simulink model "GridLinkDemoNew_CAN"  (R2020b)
settings: Solver=FixedStepDiscrete  StartTime=0.0  StopTime=inf  RelTol=1e-3  EnableMultiTasking=on
InitFcn:
  | clc
  | close all
  | f_mod = 50000;
  | f_mod1 = 50*1e3; %[12 24 36 48 72 84 96 144]*1e3; %[18 36 48 72 84 96 144]*1e3;%
  | 
  | 
  | %%
  | 
  | 
  |             Tmod1 = 1/f_mod1;
  |             Tmod = 1/f_mod;
  |             Tc = Tmod1;
  |             Tsw=Tc;
  | 
  | warning off
  | f_sig = 60;
  | 
  | U_ac = 10;
  | U_dc = 20;
  | Ts= 0.01*Tsw;
  | 
  | Fc=50000
  | Fc1=1000
  | 
  | 
  | CounterCut_Outer=2000
  | 
  | 
  | INNER_PWM=1000
  | OUTER_PWM=50000
undefined symbols (not defined in the file): A, ADCIN0, ADCIN1, ADCINA0, ADCINB0, bit, Compare, conversion, DCAEVT1, DCAEVT1FILT, Digital, Down, ended, Event, Filtered, GPTRIP1SEL, GPTRIP2SEL, hex2dec, identifier, input, Module, Newinv, of, Single, SPS_EMT_TAPAS_2018b, Standard, start, Trip, TZ1, TZ2, Up, version, Zone
libraries: tiiqmathlib x63, c2802xlib x25, c2837xDlib x5, c280xlib x5, c28xdmclib x2, svdutilitieslib x1, c2000lib x1, canmsglib x1, simulink x1
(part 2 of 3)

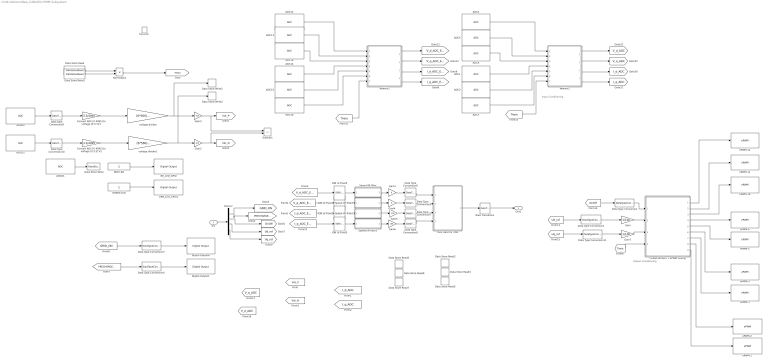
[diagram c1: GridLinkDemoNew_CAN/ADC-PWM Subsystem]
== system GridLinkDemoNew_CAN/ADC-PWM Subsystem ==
  note: Output Conditioning
  note: Input Conditioning
  In1 : Inport
  function : TriggerPort  TriggerType=function-call  VariantControl=Variant
  ADC1 : c2802xlib/ADC  blkParamProc=C2000_Type4  ADCModule=A  samplingMode=Single sample mode  ADCResolution=12-bit (Single-ended input)  useSOC1=SOC12  useSOC2=SOC0_SOC1  SOCAcquisitionWindow=13  SOCTriggerSource=ePWM12_ADCSOCA  SOCInterruptTrigger=No ADCINT  Ts=-1  dType=uint16  postInterrupt=off  interruptSel=ADCINT1  ADCINTContinuous=on  endma=off  chdma=1  conv1=ADCINA0  conv2=ADCINA0 and ADCINB0  conv1_Type4=ADCIN3  conv2_Type4=ADCIN0 and ADCIN1
  ADC12 : c2802xlib/ADC  blkParamProc=C2000_Type4  ADCModule=A  samplingMode=Single sample mode  ADCResolution=12-bit (Single-ended input)  useSOC1=SOC0  useSOC2=SOC0_SOC1  SOCAcquisitionWindow=13  SOCTriggerSource=ePWM12_ADCSOCA  SOCInterruptTrigger=No ADCINT  Ts=-1  dType=uint16  postInterrupt=off  interruptSel=ADCINT1  ADCINTContinuous=on  endma=off  chdma=1  conv1=ADCINA0  conv2=ADCINA0 and ADCINB0  conv1_Type4=ADCIN0  conv2_Type4=ADCIN0 and ADCIN1
  ADC13 : c2802xlib/ADC  blkParamProc=C2000_Type4  ADCModule=A  samplingMode=Single sample mode  ADCResolution=12-bit (Single-ended input)  useSOC1=SOC15  useSOC2=SOC0_SOC1  SOCAcquisitionWindow=13  SOCTriggerSource=ePWM12_ADCSOCA  SOCInterruptTrigger=No ADCINT  Ts=-1  dType=uint16  postInterrupt=on  interruptSel=ADCINT1  ADCINTContinuous=off  endma=off  chdma=1  conv1=ADCINA0  conv2=ADCINA0 and ADCINB0  conv1_Type4=ADCIN1  conv2_Type4=ADCIN0 and ADCIN1
  ADC14 : c2802xlib/ADC  blkParamProc=C2000_Type4  ADCModule=B  samplingMode=Single sample mode  ADCResolution=12-bit (Single-ended input)  useSOC1=SOC3  useSOC2=SOC0_SOC1  SOCAcquisitionWindow=13  SOCTriggerSource=ePWM12_ADCSOCA  SOCInterruptTrigger=No ADCINT  Ts=-1  dType=uint16  postInterrupt=off  interruptSel=ADCINT1  ADCINTContinuous=on  endma=off  chdma=1  conv1=ADCINA0  conv2=ADCINA0 and ADCINB0  conv1_Type4=ADCIN2  conv2_Type4=ADCIN0 and ADCIN1
  ADC15 : c2802xlib/ADC  blkParamProc=C2000_Type4  ADCModule=D  samplingMode=Single sample mode  ADCResolution=12-bit (Single-ended input)  useSOC1=SOC4  useSOC2=SOC0_SOC1  SOCAcquisitionWindow=13  SOCTriggerSource=ePWM12_ADCSOCA  SOCInterruptTrigger=No ADCINT  Ts=-1  dType=uint16  postInterrupt=off  interruptSel=ADCINT1  ADCINTContinuous=on  endma=off  chdma=1  conv1=ADCINA0  conv2=ADCINA0 and ADCINB0  conv1_Type4=ADCIN14  conv2_Type4=ADCIN0 and ADCIN1
  ADC16 : c2802xlib/ADC  blkParamProc=C2000_Type4  ADCModule=C  samplingMode=Single sample mode  ADCResolution=12-bit (Single-ended input)  useSOC1=SOC5  useSOC2=SOC0_SOC1  SOCAcquisitionWindow=13  SOCTriggerSource=ePWM12_ADCSOCA  SOCInterruptTrigger=No ADCINT  Ts=-1  dType=uint16  postInterrupt=off  interruptSel=ADCINT1  ADCINTContinuous=on  endma=off  chdma=1  conv1=ADCINA0  conv2=ADCINA0 and ADCINB0  conv1_Type4=ADCIN2  conv2_Type4=ADCIN0 and ADCIN1
  ADC19 : c2802xlib/ADC  blkParamProc=C2000_Type4  ADCModule=B  samplingMode=Single sample mode  ADCResolution=12-bit (Single-ended input)  useSOC1=SOC2  useSOC2=SOC0_SOC1  SOCAcquisitionWindow=13  SOCTriggerSource=ePWM12_ADCSOCA  SOCInterruptTrigger=No ADCINT  Ts=-1  dType=uint16  postInterrupt=off  interruptSel=ADCINT1  ADCINTContinuous=on  endma=off  chdma=1  conv1=ADCINA0  conv2=ADCINA0 and ADCINB0  conv1_Type4=ADCIN1  conv2_Type4=ADCIN0 and ADCIN1
  ADC2 : c2802xlib/ADC  blkParamProc=C2000_Type4  ADCModule=B  samplingMode=Single sample mode  ADCResolution=12-bit (Single-ended input)  useSOC1=SOC13  useSOC2=SOC0_SOC1  SOCAcquisitionWindow=13  SOCTriggerSource=ePWM12_ADCSOCA  SOCInterruptTrigger=No ADCINT  Ts=-1  dType=uint16  postInterrupt=off  interruptSel=ADCINT1  ADCINTContinuous=on  endma=off  chdma=1  conv1=ADCINA0  conv2=ADCINA0 and ADCINB0  conv1_Type4=ADCIN0  conv2_Type4=ADCIN0 and ADCIN1
  ADC3 : c2802xlib/ADC  blkParamProc=C2000_Type4  ADCModule=D  samplingMode=Single sample mode  ADCResolution=12-bit (Single-ended input)  useSOC1=SOC2  useSOC2=SOC0_SOC1  SOCAcquisitionWindow=13  SOCTriggerSource=ePWM12_ADCSOCA  SOCInterruptTrigger=No ADCINT  Ts=-1  dType=uint16  postInterrupt=off  interruptSel=ADCINT1  ADCINTContinuous=off  endma=off  chdma=1  conv1=ADCINA0  conv2=ADCINA0 and ADCINB0  conv1_Type4=ADCIN4  conv2_Type4=ADCIN0 and ADCIN1
  ADC4 : c2802xlib/ADC  blkParamProc=C2000_Type4  ADCModule=A  samplingMode=Single sample mode  ADCResolution=12-bit (Single-ended input)  useSOC1=SOC9  useSOC2=SOC0_SOC1  SOCAcquisitionWindow=13  SOCTriggerSource=ePWM12_ADCSOCA  SOCInterruptTrigger=No ADCINT  Ts=-1  dType=uint16  postInterrupt=off  interruptSel=ADCINT1  ADCINTContinuous=on  endma=off  chdma=1  conv1=ADCINA0  conv2=ADCINA0 and ADCINB0  conv1_Type4=ADCIN5  conv2_Type4=ADCIN0 and ADCIN1
  ADC5 : c2802xlib/ADC  blkParamProc=C2000_Type4  ADCModule=B  samplingMode=Single sample mode  ADCResolution=12-bit (Single-ended input)  useSOC1=SOC10  useSOC2=SOC0_SOC1  SOCAcquisitionWindow=13  SOCTriggerSource=ePWM12_ADCSOCA  SOCInterruptTrigger=No ADCINT  Ts=-1  dType=uint16  postInterrupt=off  interruptSel=ADCINT1  ADCINTContinuous=on  endma=off  chdma=1  conv1=ADCINA0  conv2=ADCINA0 and ADCINB0  conv1_Type4=ADCIN4  conv2_Type4=ADCIN0 and ADCIN1
  ADC6 : c2802xlib/ADC  blkParamProc=C2000_Type4  ADCModule=D  samplingMode=Single sample mode  ADCResolution=12-bit (Single-ended input)  useSOC1=SOC11  useSOC2=SOC0_SOC1  SOCAcquisitionWindow=13  SOCTriggerSource=ePWM12_ADCSOCA  SOCInterruptTrigger=No ADCINT  Ts=-1  dType=uint16  postInterrupt=off  interruptSel=ADCINT1  ADCINTContinuous=on  endma=off  chdma=1  conv1=ADCINA0  conv2=ADCINA0 and ADCINB0  conv1_Type4=ADCIN5  conv2_Type4=ADCIN0 and ADCIN1
  ADCD0 : c2802xlib/ADC  blkParamProc=C2000_Type4  ADCModule=D  samplingMode=Single sample mode  ADCResolution=12-bit (Single-ended input)  useSOC1=SOC6  useSOC2=SOC0_SOC1  SOCAcquisitionWindow=13  SOCTriggerSource=ePWM12_ADCSOCA  SOCInterruptTrigger=No ADCINT  Ts=-1  dType=uint16  postInterrupt=off  interruptSel=ADCINT1  ADCINTContinuous=off  endma=off  chdma=1  conv1=ADCINA0  conv2=ADCINA0 and ADCINB0  conv1_Type4=ADCIN0  conv2_Type4=ADCIN0 and ADCIN1
  ADCD1 : c2802xlib/ADC  blkParamProc=C2000_Type4  ADCModule=D  samplingMode=Single sample mode  ADCResolution=12-bit (Single-ended input)  useSOC1=SOC7  useSOC2=SOC0_SOC1  SOCAcquisitionWindow=13  SOCTriggerSource=ePWM12_ADCSOCA  SOCInterruptTrigger=No ADCINT  Ts=-1  dType=uint16  postInterrupt=off  interruptSel=ADCINT1  ADCINTContinuous=off  endma=off  chdma=1  conv1=ADCINA0  conv2=ADCINA0 and ADCINB0  conv1_Type4=ADCIN1  conv2_Type4=ADCIN0 and ADCIN1
  ADCD2 : c2802xlib/ADC  blkParamProc=C2000_Type4  ADCModule=D  samplingMode=Single sample mode  ADCResolution=12-bit (Single-ended input)  useSOC1=SOC8  useSOC2=SOC0_SOC1  SOCAcquisitionWindow=13  SOCTriggerSource=ePWM12_ADCSOCA  SOCInterruptTrigger=No ADCINT  Ts=-1  dType=uint16  postInterrupt=off  interruptSel=ADCINT2  ADCINTContinuous=off  endma=off  chdma=1  conv1=ADCINA0  conv2=ADCINA0 and ADCINB0  conv1_Type4=ADCIN2  conv2_Type4=ADCIN0 and ADCIN1
  Convert ADC [0 4095] to voltage [0 3.3] V : Gain  Gain=3.3/4095  ParamDataTypeStr=Inherit: Inherit from 'Gain'  OutDataTypeStr=single
  Convert ADC [0 4095] to voltage [0 3.3] V1 : Gain  Gain=3.3/4095  ParamDataTypeStr=Inherit: Inherit from 'Gain'  OutDataTypeStr=single
  Data Store Read : DataStoreRead  DataStoreName=Counter
  Data Store Read1 : DataStoreRead  DataStoreName=CounterCut
  Data Store Read2 : DataStoreRead  DataStoreName=I_o_C
  Data Store Read3 : DataStoreRead  DataStoreName=I_s_C
  Data Store Read4 : DataStoreRead  DataStoreName=I_s_B
  Data Store Read5 : DataStoreRead  DataStoreName=I_s_A
  Data Store Read6 : DataStoreRead  DataStoreName=I_o_B
  Data Store Read7 : DataStoreRead  DataStoreName=I_o_A
  Data Store Write : DataStoreWrite  DataStoreName=Temp_P1
  Data Store Write1 : DataStoreWrite  DataStoreName=VdcP
  Data Store Write2 : DataStoreWrite  DataStoreName=VdcN
  Data Type Conversion : DataTypeConversion  OutDataTypeStr=boolean
  Data Type Conversion{1,5..11} (8 alike) : DataTypeConversion  OutDataTypeStr=single
  Data Type Conversion3 : DataTypeConversion  OutDataTypeStr=boolean
  Data Type Conversion4 : DataTypeConversion  OutDataTypeStr=boolean
  Demux : Demux
  Digital Output1 : c2837xDlib/Digital Output  GPIO_Number=GPIO64~GPIO71  GPIO_Bit0=off  GPIO_BIT0_Toggle=on  GPIO_Bit1=off  GPIO_BIT1_Toggle=on  GPIO_Bit2=off  GPIO_BIT2_Toggle=off  GPIO_Bit3=off  GPIO_BIT3_Toggle=off  GPIO_Bit4=off  GPIO_BIT4_Toggle=off  GPIO_Bit5=off  GPIO_BIT5_Toggle=off  GPIO_Bit6=off  GPIO_BIT6_Toggle=off  GPIO_Bit7=on  GPIO_BIT7_Toggle=off
  Digital Output6 : c2837xDlib/Digital Output  GPIO_Number=GPIO56~GPIO63  GPIO_Bit0=off  GPIO_BIT0_Toggle=off  GPIO_Bit1=on  GPIO_BIT1_Toggle=off  GPIO_Bit2=off  GPIO_BIT2_Toggle=off  GPIO_Bit3=off  GPIO_BIT3_Toggle=off  GPIO_Bit4=off  GPIO_BIT4_Toggle=off  GPIO_Bit5=off  GPIO_BIT5_Toggle=on  GPIO_Bit6=off  GPIO_BIT6_Toggle=off  GPIO_Bit7=off  GPIO_BIT7_Toggle=on
  GREEN LED : Constant  OutDataTypeStr=boolean  SampleTime=-1
  GRN_LED_GPIO1 : c2837xDlib/Digital Output  GPIO_Number=GPIO112~GPIO119  GPIO_Bit0=off  GPIO_BIT0_Toggle=on  GPIO_Bit1=off  GPIO_BIT1_Toggle=on  GPIO_Bit2=on  GPIO_BIT2_Toggle=off  GPIO_Bit3=off  GPIO_BIT3_Toggle=off  GPIO_Bit4=off  GPIO_BIT4_Toggle=off  GPIO_Bit5=off  GPIO_BIT5_Toggle=on  GPIO_Bit6=off  GPIO_BIT6_Toggle=off  GPIO_Bit7=off  GPIO_BIT7_Toggle=on
  Gain : Gain  Gain=1/100
  Gain1 : Gain
  Gain2 : Gain  Gain=100  ParamDataTypeStr=Inherit: Inherit from 'Gain'
  Gain3 : Gain  Gain=100  ParamDataTypeStr=Inherit: Inherit from 'Gain'
  Gain4 : Gain
  Gain5 : Gain  Gain=100
  Gain6 : Gain  Gain=100
  Gain7 : Gain  Gain=1/100
  IQN to Float{1..3,5} (4 alike) : tiiqmathlib/IQN to Float
  InvPark/SVGen + ePWM scaling : Subsystem
  Newinv1 : Subsystem  AncestorBlock=SPS_EMT_TAPAS_2018b/Newinv  TreatAsAtomicUnit=on
  Newinv2 : Subsystem  AncestorBlock=SPS_EMT_TAPAS_2018b/Newinv  TreatAsAtomicUnit=on
  Normalize1 : Product  Inputs=*/
  Pack data for CAN : Subsystem
  RD_LED_GPIO : c2837xDlib/Digital Output  GPIO_Number=GPIO112~GPIO119  GPIO_Bit0=off  GPIO_BIT0_Toggle=on  GPIO_Bit1=on  GPIO_BIT1_Toggle=off  GPIO_Bit2=off  GPIO_BIT2_Toggle=on  GPIO_Bit3=off  GPIO_BIT3_Toggle=off  GPIO_Bit4=off  GPIO_BIT4_Toggle=off  GPIO_Bit5=off  GPIO_BIT5_Toggle=off  GPIO_Bit6=off  GPIO_BIT6_Toggle=on  GPIO_Bit7=off  GPIO_BIT7_Toggle=on
  RED LED : Constant  OutDataTypeStr=boolean  SampleTime=-1
  Rate Transition1 : RateTransition
  Speed IIR filter : Subsystem
  Speed IIR filter1 : Subsystem
  Speed IIR filter2 : Subsystem
  Speed IIR filter3 : Subsystem
  Subtract : Sum  Inputs=+-
  "ePWM-1 " : c2802xlib/ePWM  PwmType=C2000_Type4  useModule=ePWM1  ePWMxLINKTBPRD=Not Linked  periodUnits=Clock cycles  timerSource=Specify via dialog  timerPeriod_clk=INNER_PWM  timerPeriod_sec=0.0001  tbshadow=Counter equals to zero  countingMode=Up-Down  phaseActiveEnable=Set counter to phase value specified via dialog  phaseDirection=Count up after sync  phaseActive=0  synchronizationEnable=off  dcaevt1Sync=off  dcbevt1Sync=off  synchronizationOption=Disable  perSynchronizationOption=Counter equals to period (CTR=PRD)  clockPrescale=1  HSclockPrescale=1  enswap=off  ePWMxAStatus=on  ePWMxAactionLogic1=Do nothing  ePWMxAactionLogic2=Do nothing  ePWMxAactionLogic3=Clear  ePWMxAactionLogic4=Set  ePWMxAactionLogic5=Do nothing  ePWMxAactionLogic6=Do nothing  ePWMxACSFenable=off  ePWMxACSFvalue=Forcing disable  ePWMxASFreload=Immediate  ePWMxBStatus=off  ePWMxBactionLogic1=Do nothing  ePWMxBactionLogic2=Do nothing  ePWMxBactionLogic3=Clear  ePWMxBactionLogic4=Set  ePWMxBactionLogic5=Do nothing  ePWMxBactionLogic6=Do nothing  ePWMxBCSFenable=off  ePWMxBCSFvalue=Forcing disable  ePWMxBSFreload=Immediate  ePWNxBOutWay=off  ePWMxLINKCMPA=Not Linked  CMPAUnits=Clock cycles  CMPASource=Input port  CMPAValue_per=50  CMPAValue_clk=0  enCMPAshadow=Counter equals to zero (CTR=Zero)  ePWMxLINKCMPB=Not Linked  CMPBUnits=Clock cycles  CMPBSource=Specify via dialog  CMPBValue_per=50  CMPBValue_clk=32000  enCMPBshadow=Counter equals to zero (CTR=Zero)  ePWMxLINKCMPC=Not Linked  CMPCUnits=Clock cycles  CMPCSource=Specify via dialog  CMPCValue_per=50  CMPCValue_clk=32000  enCMPCshadow=Counter equals to zero (CTR=Zero)  ePWMxLINKCMPD=Not Linked  CMPDUnits=Clock cycles  CMPDSource=Specify via dialog  CMPDValue_per=50  CMPDValue_clk=32000  enCMPDshadow=Counter equals to zero (CTR=Zero)  enableDBePWMxA=on  enableDBePWMxB=on  enhalfcycle=off  DBpolarity=Active high complementary (AHC)  DBedgeDelay=Positive  DBSource_ePWMxA=ePWMxA  DBSource_ePWMxB=ePWMxA  DBPeriodUnits=Clock cycles  DBperiodSource=Specify via dialog  REDperiod=2  FEDperiod=2  REDperiod_sec=0  FEDperiod_sec=0  LoadModeDBRED=Immediate without using shadow  LoadModeDBFED=Immediate without using shadow  adcstartModuleA=off  adcrequestEventA=First event  adcstartEventA=Digital Compare Module A Event 1 start of conversion (DCAEVT1.soc)  adcstartEventA_type2=Counter equals to period (CTR=PRD)  adcstartModuleB=off  adcrequestEventB=First event  adcstartEventB=Counter equals to zero (CTR=Zero)  adcstartEventB_type2=Counter equals to zero (CTR=Zero)  intEn=off  intPrd=First event  intSel=Counter equals to zero (CTR=Zero)  intSel_type2=Counter equals to zero (CTR=Zero)  hrpe=off  enHRPWM=off  HRPWM_LoadMode=Counter equals to period (CTR=PRD)  HRPWM_CTLMode=Duty or Period control mode  HRPWM_EDGMode=Both edge  hrpeb=off  enHRPWMB=off  HRPWM_LoadModeB=Counter equals to zero (CTR=ZERO)  HRPWM_CTLModeB=Duty or Period control mode  HRPWM_EDGModeB=Both edge  enHRDBRED=off  enHRDBFED=off  enSFO=on  enautoconv=on  chopperEnable=off  chopperFrequency=1  chopperFirstwidth=1  chopperDuty=12.5%  tripZonesource=Specify via dialog  tzselOSHT1=off  tzselOSHT2=off  tzselOSHT3=off  tzselOSHDCAEV1=off  tzselOSHDCBEV1=off  tzselCBC1=off  tzselCBC2=off  tzselCBC3=off  tzselCBCDCAEV2=off  tzselCBCDCBEV2=off  tzselOSHT4=off  tzselOSHT5=off  tzselOSHT6=off  tzselCBC4=off  tzselCBC5=off  tzselCBC6=off  enTzOstIntr=off  enTzCbcIntr=off  enTzDCAEVT1Intr=off  enTzDCAEVT2Intr=off  enTzDCBEVT1Intr=off  enTzDCBEVT2Intr=off  ePWMxAforced=No action  ePWMxBforced=No action  DCAEVT1forced=No action  DCBEVT1forced=No action  DCAEVT2forced=No action  DCBEVT2forced=No action  dcah=Trip Zone 1 input (TZ1)  dcal=Trip Zone 2 input (TZ2)  dcbh=Trip Zone 1 input (TZ1)  dcbl=Trip Zone 2 input (TZ2)  dcah_type2=GPTRIP1SEL/(TZ1)  dcal_type2=GPTRIP2SEL/(TZ2)  dcbh_type2=GPTRIP1SEL/(TZ1)  dcbl_type2=GPTRIP2SEL/(TZ2)  gendcaevt1=Event disabled  gendcaevt2=Event disabled  gendcbevt1=Event disabled  gendcbevt2=Event disabled  dcaevt1src=DCAEVT1 with sync  dcaevt2src=DCAEVT2 with sync  dcbevt1src=DCBEVT1 with sync  dcbevt2src=DCBEVT2 with sync  pulsesel=Counter equals to zero (CTR=Zero)  blankinv=off  blankoffset=0  blankwidth=0  evsrcsel=Filtered version of DCAEVT1 (DCAEVT1FILT)  encape=off
  ePWM-10 : c2802xlib/ePWM  PwmType=C2000_Type4  useModule=ePWM10  ePWMxLINKTBPRD=Not Linked  periodUnits=Clock cycles  timerSource=Specify via dialog  timerPeriod_clk=OUTER_PWM  timerPeriod_sec=0.0001  tbshadow=Counter equals to zero  countingMode=Up-Down  phaseActiveEnable=Set counter to phase value specified via dialog  phaseDirection=Count up after sync  phaseActive=0  synchronizationEnable=off  dcaevt1Sync=off  dcbevt1Sync=off  synchronizationOption=Disable  perSynchronizationOption=Counter equals to period (CTR=PRD)  clockPrescale=1  HSclockPrescale=1  enswap=off  ePWMxAStatus=on  ePWMxAactionLogic1=Do nothing  ePWMxAactionLogic2=Do nothing  ePWMxAactionLogic3=Clear  ePWMxAactionLogic4=Set  ePWMxAactionLogic5=Do nothing  ePWMxAactionLogic6=Do nothing  ePWMxACSFenable=off  ePWMxACSFvalue=Forcing disable  ePWMxASFreload=Immediate  ePWMxBStatus=off  ePWMxBactionLogic1=Do nothing  ePWMxBactionLogic2=Do nothing  ePWMxBactionLogic3=Clear  ePWMxBactionLogic4=Set  ePWMxBactionLogic5=Do nothing  ePWMxBactionLogic6=Do nothing  ePWMxBCSFenable=off  ePWMxBCSFvalue=Forcing disable  ePWMxBSFreload=Immediate  ePWNxBOutWay=off  ePWMxLINKCMPA=Not Linked  CMPAUnits=Clock cycles  CMPASource=Input port  CMPAValue_per=50  CMPAValue_clk=0  enCMPAshadow=Counter equals to zero (CTR=Zero)  ePWMxLINKCMPB=Not Linked  CMPBUnits=Clock cycles  CMPBSource=Specify via dialog  CMPBValue_per=50  CMPBValue_clk=32000  enCMPBshadow=Counter equals to zero (CTR=Zero)  ePWMxLINKCMPC=Not Linked  CMPCUnits=Clock cycles  CMPCSource=Specify via dialog  CMPCValue_per=50  CMPCValue_clk=32000  enCMPCshadow=Counter equals to zero (CTR=Zero)  ePWMxLINKCMPD=Not Linked  CMPDUnits=Clock cycles  CMPDSource=Specify via dialog  CMPDValue_per=50  CMPDValue_clk=32000  enCMPDshadow=Counter equals to zero (CTR=Zero)  enableDBePWMxA=on  enableDBePWMxB=on  enhalfcycle=off  DBpolarity=Active high complementary (AHC)  DBedgeDelay=Positive  DBSource_ePWMxA=ePWMxA  DBSource_ePWMxB=ePWMxA  DBPeriodUnits=Clock cycles  DBperiodSource=Specify via dialog  REDperiod=25  FEDperiod=25  REDperiod_sec=0  FEDperiod_sec=0  LoadModeDBRED=Immediate without using shadow  LoadModeDBFED=Immediate without using shadow  adcstartModuleA=off  adcrequestEventA=First event  adcstartEventA=Digital Compare Module A Event 1 start of conversion (DCAEVT1.soc)  adcstartEventA_type2=Counter equals to period (CTR=PRD)  adcstartModuleB=off  adcrequestEventB=First event  adcstartEventB=Counter equals to zero (CTR=Zero)  adcstartEventB_type2=Counter equals to zero (CTR=Zero)  intEn=off  intPrd=First event  intSel=Counter equals to zero (CTR=Zero)  intSel_type2=Counter equals to zero (CTR=Zero)  hrpe=off  enHRPWM=off  HRPWM_LoadMode=Counter equals to period (CTR=PRD)  HRPWM_CTLMode=Duty or Period control mode  HRPWM_EDGMode=Both edge  hrpeb=off  enHRPWMB=off  HRPWM_LoadModeB=Counter equals to zero (CTR=ZERO)  HRPWM_CTLModeB=Duty or Period control mode  HRPWM_EDGModeB=Both edge  enHRDBRED=off  enHRDBFED=off  enSFO=on  enautoconv=on  chopperEnable=off  chopperFrequency=1  chopperFirstwidth=1  chopperDuty=12.5%  tripZonesource=Specify via dialog  tzselOSHT1=off  tzselOSHT2=off  tzselOSHT3=off  tzselOSHDCAEV1=off  tzselOSHDCBEV1=off  tzselCBC1=off  tzselCBC2=off  tzselCBC3=off  tzselCBCDCAEV2=off  tzselCBCDCBEV2=off  tzselOSHT4=off  tzselOSHT5=off  tzselOSHT6=off  tzselCBC4=off  tzselCBC5=off  tzselCBC6=off  enTzOstIntr=off  enTzCbcIntr=off  enTzDCAEVT1Intr=off  enTzDCAEVT2Intr=off  enTzDCBEVT1Intr=off  enTzDCBEVT2Intr=off  ePWMxAforced=No action  ePWMxBforced=No action  DCAEVT1forced=No action  DCBEVT1forced=No action  DCAEVT2forced=No action  DCBEVT2forced=No action  dcah=Trip Zone 1 input (TZ1)  dcal=Trip Zone 2 input (TZ2)  dcbh=Trip Zone 1 input (TZ1)  dcbl=Trip Zone 2 input (TZ2)  dcah_type2=GPTRIP1SEL/(TZ1)  dcal_type2=GPTRIP2SEL/(TZ2)  dcbh_type2=GPTRIP1SEL/(TZ1)  dcbl_type2=GPTRIP2SEL/(TZ2)  gendcaevt1=Event disabled  gendcaevt2=Event disabled  gendcbevt1=Event disabled  gendcbevt2=Event disabled  dcaevt1src=DCAEVT1 with sync  dcaevt2src=DCAEVT2 with sync  dcbevt1src=DCBEVT1 with sync  dcbevt2src=DCBEVT2 with sync  pulsesel=Counter equals to zero (CTR=Zero)  blankinv=off  blankoffset=0  blankwidth=0  evsrcsel=Filtered version of DCAEVT1 (DCAEVT1FILT)  encape=off
  ePWM-11 : c2802xlib/ePWM  PwmType=C2000_Type4  useModule=ePWM11  ePWMxLINKTBPRD=Not Linked  periodUnits=Clock cycles  timerSource=Specify via dialog  timerPeriod_clk=OUTER_PWM  timerPeriod_sec=0.0001  tbshadow=Counter equals to zero  countingMode=Up-Down  phaseActiveEnable=Set counter to phase value specified via dialog  phaseDirection=Count up after sync  phaseActive=0  synchronizationEnable=off  dcaevt1Sync=off  dcbevt1Sync=off  synchronizationOption=Pass through (EPWMxSYNCI or SWFSYNC)  perSynchronizationOption=Counter equals to period (CTR=PRD)  clockPrescale=1  HSclockPrescale=1  enswap=off  ePWMxAStatus=on  ePWMxAactionLogic1=Do nothing  ePWMxAactionLogic2=Do nothing  ePWMxAactionLogic3=Clear  ePWMxAactionLogic4=Set  ePWMxAactionLogic5=Do nothing  ePWMxAactionLogic6=Do nothing  ePWMxACSFenable=off  ePWMxACSFvalue=Forcing disable  ePWMxASFreload=Immediate  ePWMxBStatus=off  ePWMxBactionLogic1=Do nothing  ePWMxBactionLogic2=Do nothing  ePWMxBactionLogic3=Clear  ePWMxBactionLogic4=Set  ePWMxBactionLogic5=Do nothing  ePWMxBactionLogic6=Do nothing  ePWMxBCSFenable=off  ePWMxBCSFvalue=Forcing disable  ePWMxBSFreload=Immediate  ePWNxBOutWay=off  ePWMxLINKCMPA=Not Linked  CMPAUnits=Clock cycles  CMPASource=Input port  CMPAValue_per=50  CMPAValue_clk=0  enCMPAshadow=Counter equals to zero (CTR=Zero)  ePWMxLINKCMPB=Not Linked  CMPBUnits=Clock cycles  CMPBSource=Specify via dialog  CMPBValue_per=50  CMPBValue_clk=32000  enCMPBshadow=Counter equals to zero (CTR=Zero)  ePWMxLINKCMPC=Not Linked  CMPCUnits=Clock cycles  CMPCSource=Specify via dialog  CMPCValue_per=50  CMPCValue_clk=32000  enCMPCshadow=Counter equals to zero (CTR=Zero)  ePWMxLINKCMPD=Not Linked  CMPDUnits=Clock cycles  CMPDSource=Specify via dialog  CMPDValue_per=50  CMPDValue_clk=32000  enCMPDshadow=Counter equals to zero (CTR=Zero)  enableDBePWMxA=on  enableDBePWMxB=on  enhalfcycle=off  DBpolarity=Active high complementary (AHC)  DBedgeDelay=Positive  DBSource_ePWMxA=ePWMxA  DBSource_ePWMxB=ePWMxA  DBPeriodUnits=Clock cycles  DBperiodSource=Specify via dialog  REDperiod=25  FEDperiod=25  REDperiod_sec=0  FEDperiod_sec=0  LoadModeDBRED=Immediate without using shadow  LoadModeDBFED=Immediate without using shadow  adcstartModuleA=off  adcrequestEventA=First event  adcstartEventA=Digital Compare Module A Event 1 start of conversion (DCAEVT1.soc)  adcstartEventA_type2=Counter equals to period (CTR=PRD)  adcstartModuleB=off  adcrequestEventB=First event  adcstartEventB=Counter equals to zero (CTR=Zero)  adcstartEventB_type2=Counter equals to zero (CTR=Zero)  intEn=off  intPrd=First event  intSel=Counter equals to zero (CTR=Zero)  intSel_type2=Counter equals to zero (CTR=Zero)  hrpe=off  enHRPWM=off  HRPWM_LoadMode=Counter equals to period (CTR=PRD)  HRPWM_CTLMode=Duty or Period control mode  HRPWM_EDGMode=Both edge  hrpeb=off  enHRPWMB=off  HRPWM_LoadModeB=Counter equals to zero (CTR=ZERO)  HRPWM_CTLModeB=Duty or Period control mode  HRPWM_EDGModeB=Both edge  enHRDBRED=off  enHRDBFED=off  enSFO=on  enautoconv=on  chopperEnable=off  chopperFrequency=1  chopperFirstwidth=1  chopperDuty=12.5%  tripZonesource=Specify via dialog  tzselOSHT1=off  tzselOSHT2=off  tzselOSHT3=off  tzselOSHDCAEV1=off  tzselOSHDCBEV1=off  tzselCBC1=off  tzselCBC2=off  tzselCBC3=off  tzselCBCDCAEV2=off  tzselCBCDCBEV2=off  tzselOSHT4=off  tzselOSHT5=off  tzselOSHT6=off  tzselCBC4=off  tzselCBC5=off  tzselCBC6=off  enTzOstIntr=off  enTzCbcIntr=off  enTzDCAEVT1Intr=off  enTzDCAEVT2Intr=off  enTzDCBEVT1Intr=off  enTzDCBEVT2Intr=off  ePWMxAforced=No action  ePWMxBforced=No action  DCAEVT1forced=No action  DCBEVT1forced=No action  DCAEVT2forced=No action  DCBEVT2forced=No action  dcah=Trip Zone 1 input (TZ1)  dcal=Trip Zone 2 input (TZ2)  dcbh=Trip Zone 1 input (TZ1)  dcbl=Trip Zone 2 input (TZ2)  dcah_type2=GPTRIP1SEL/(TZ1)  dcal_type2=GPTRIP2SEL/(TZ2)  dcbh_type2=GPTRIP1SEL/(TZ1)  dcbl_type2=GPTRIP2SEL/(TZ2)  gendcaevt1=Event disabled  gendcaevt2=Event disabled  gendcbevt1=Event disabled  gendcbevt2=Event disabled  dcaevt1src=DCAEVT1 with sync  dcaevt2src=DCAEVT2 with sync  dcbevt1src=DCBEVT1 with sync  dcbevt2src=DCBEVT2 with sync  pulsesel=Counter equals to zero (CTR=Zero)  blankinv=off  blankoffset=0  blankwidth=0  evsrcsel=Filtered version of DCAEVT1 (DCAEVT1FILT)  encape=off
  ePWM-12 : c2802xlib/ePWM  PwmType=C2000_Type4  useModule=ePWM12  ePWMxLINKTBPRD=Not Linked  periodUnits=Clock cycles  timerSource=Specify via dialog  timerPeriod_clk=OUTER_PWM  timerPeriod_sec=0.0001  tbshadow=Counter equals to zero  countingMode=Up-Down  phaseActiveEnable=Disable  phaseDirection=Count down after sync  phaseActive=0  synchronizationEnable=off  dcaevt1Sync=off  dcbevt1Sync=off  synchronizationOption=Counter equals to zero (CTR=Zero)  perSynchronizationOption=Counter equals to period (CTR=PRD)  clockPrescale=1  HSclockPrescale=1  enswap=off  ePWMxAStatus=on  ePWMxAactionLogic1=Do nothing  ePWMxAactionLogic2=Do nothing  ePWMxAactionLogic3=Clear  ePWMxAactionLogic4=Set  ePWMxAactionLogic5=Do nothing  ePWMxAactionLogic6=Do nothing  ePWMxACSFenable=off  ePWMxACSFvalue=Forcing disable  ePWMxASFreload=Immediate  ePWMxBStatus=off  ePWMxBactionLogic1=Do nothing  ePWMxBactionLogic2=Do nothing  ePWMxBactionLogic3=Clear  ePWMxBactionLogic4=Set  ePWMxBactionLogic5=Do nothing  ePWMxBactionLogic6=Do nothing  ePWMxBCSFenable=off  ePWMxBCSFvalue=Forcing disable  ePWMxBSFreload=Immediate  ePWNxBOutWay=off  ePWMxLINKCMPA=Not Linked  CMPAUnits=Clock cycles  CMPASource=Input port  CMPAValue_per=50  CMPAValue_clk=0  enCMPAshadow=Counter equals to zero (CTR=Zero)  ePWMxLINKCMPB=Not Linked  CMPBUnits=Clock cycles  CMPBSource=Specify via dialog  CMPBValue_per=50  CMPBValue_clk=32000  enCMPBshadow=Counter equals to zero (CTR=Zero)  ePWMxLINKCMPC=Not Linked  CMPCUnits=Clock cycles  CMPCSource=Specify via dialog  CMPCValue_per=50  CMPCValue_clk=32000  enCMPCshadow=Counter equals to zero (CTR=Zero)  ePWMxLINKCMPD=Not Linked  CMPDUnits=Clock cycles  CMPDSource=Specify via dialog  CMPDValue_per=50  CMPDValue_clk=32000  enCMPDshadow=Counter equals to zero (CTR=Zero)  enableDBePWMxA=on  enableDBePWMxB=on  enhalfcycle=on  DBpolarity=Active high complementary (AHC)  DBedgeDelay=Positive  DBSource_ePWMxA=ePWMxA  DBSource_ePWMxB=ePWMxA  DBPeriodUnits=Clock cycles  DBperiodSource=Specify via dialog  REDperiod=25  FEDperiod=25  REDperiod_sec=0  FEDperiod_sec=0  LoadModeDBRED=Immediate without using shadow  LoadModeDBFED=Immediate without using shadow  adcstartModuleA=on  adcrequestEventA=First event  adcstartEventA=Digital Compare Module A Event 1 start of conversion (DCAEVT1.soc)  adcstartEventA_type2=Counter equals to period (CTR=PRD)  adcstartModuleB=off  adcrequestEventB=First event  adcstartEventB=Counter equals to zero (CTR=Zero)  adcstartEventB_type2=Counter equals to zero (CTR=Zero)  intEn=off  intPrd=First event  intSel=Counter equals to zero (CTR=Zero)  intSel_type2=Counter equals to zero (CTR=Zero)  hrpe=off  enHRPWM=off  HRPWM_LoadMode=Counter equals to period (CTR=PRD)  HRPWM_CTLMode=Duty or Period control mode  HRPWM_EDGMode=Both edge  hrpeb=off  enHRPWMB=off  HRPWM_LoadModeB=Counter equals to zero (CTR=ZERO)  HRPWM_CTLModeB=Duty or Period control mode  HRPWM_EDGModeB=Both edge  enHRDBRED=off  enHRDBFED=off  enSFO=on  enautoconv=on  chopperEnable=off  chopperFrequency=1  chopperFirstwidth=1  chopperDuty=12.5%  tripZonesource=Specify via dialog  tzselOSHT1=off  tzselOSHT2=off  tzselOSHT3=off  tzselOSHDCAEV1=off  tzselOSHDCBEV1=off  tzselCBC1=off  tzselCBC2=off  tzselCBC3=off  tzselCBCDCAEV2=off  tzselCBCDCBEV2=off  tzselOSHT4=off  tzselOSHT5=off  tzselOSHT6=off  tzselCBC4=off  tzselCBC5=off  tzselCBC6=off  enTzOstIntr=off  enTzCbcIntr=off  enTzDCAEVT1Intr=off  enTzDCAEVT2Intr=off  enTzDCBEVT1Intr=off  enTzDCBEVT2Intr=off  ePWMxAforced=No action  ePWMxBforced=No action  DCAEVT1forced=No action  DCBEVT1forced=No action  DCAEVT2forced=No action  DCBEVT2forced=No action  dcah=Trip Zone 1 input (TZ1)  dcal=Trip Zone 2 input (TZ2)  dcbh=Trip Zone 1 input (TZ1)  dcbl=Trip Zone 2 input (TZ2)  dcah_type2=GPTRIP1SEL/(TZ1)  dcal_type2=GPTRIP2SEL/(TZ2)  dcbh_type2=GPTRIP1SEL/(TZ1)  dcbl_type2=GPTRIP2SEL/(TZ2)  gendcaevt1=Event disabled  gendcaevt2=Event disabled  gendcbevt1=Event disabled  gendcbevt2=Event disabled  dcaevt1src=DCAEVT1 with sync  dcaevt2src=DCAEVT2 with sync  dcbevt1src=DCBEVT1 with sync  dcbevt2src=DCBEVT2 with sync  pulsesel=Counter equals to zero (CTR=Zero)  blankinv=off  blankoffset=0  blankwidth=0  evsrcsel=Filtered version of DCAEVT1 (DCAEVT1FILT)  encape=off
  "ePWM-2 " : c2802xlib/ePWM  PwmType=C2000_Type4  useModule=ePWM2  ePWMxLINKTBPRD=Not Linked  periodUnits=Clock cycles  timerSource=Specify via dialog  timerPeriod_clk=INNER_PWM  timerPeriod_sec=0.0001  tbshadow=Counter equals to zero  countingMode=Up-Down  phaseActiveEnable=Set counter to phase value specified via dialog  phaseDirection=Count up after sync  phaseActive=0  synchronizationEnable=off  dcaevt1Sync=off  dcbevt1Sync=off  synchronizationOption=Disable  perSynchronizationOption=Counter equals to period (CTR=PRD)  clockPrescale=1  HSclockPrescale=1  enswap=off  ePWMxAStatus=on  ePWMxAactionLogic1=Do nothing  ePWMxAactionLogic2=Do nothing  ePWMxAactionLogic3=Clear  ePWMxAactionLogic4=Set  ePWMxAactionLogic5=Do nothing  ePWMxAactionLogic6=Do nothing  ePWMxACSFenable=off  ePWMxACSFvalue=Forcing disable  ePWMxASFreload=Immediate  ePWMxBStatus=off  ePWMxBactionLogic1=Do nothing  ePWMxBactionLogic2=Do nothing  ePWMxBactionLogic3=Clear  ePWMxBactionLogic4=Set  ePWMxBactionLogic5=Do nothing  ePWMxBactionLogic6=Do nothing  ePWMxBCSFenable=off  ePWMxBCSFvalue=Forcing disable  ePWMxBSFreload=Immediate  ePWNxBOutWay=off  ePWMxLINKCMPA=Not Linked  CMPAUnits=Clock cycles  CMPASource=Input port  CMPAValue_per=50  CMPAValue_clk=0  enCMPAshadow=Counter equals to zero (CTR=Zero)  ePWMxLINKCMPB=Not Linked  CMPBUnits=Clock cycles  CMPBSource=Specify via dialog  CMPBValue_per=50  CMPBValue_clk=32000  enCMPBshadow=Counter equals to zero (CTR=Zero)  ePWMxLINKCMPC=Not Linked  CMPCUnits=Clock cycles  CMPCSource=Specify via dialog  CMPCValue_per=50  CMPCValue_clk=32000  enCMPCshadow=Counter equals to zero (CTR=Zero)  ePWMxLINKCMPD=Not Linked  CMPDUnits=Clock cycles  CMPDSource=Specify via dialog  CMPDValue_per=50  CMPDValue_clk=32000  enCMPDshadow=Counter equals to zero (CTR=Zero)  enableDBePWMxA=on  enableDBePWMxB=on  enhalfcycle=off  DBpolarity=Active high complementary (AHC)  DBedgeDelay=Positive  DBSource_ePWMxA=ePWMxA  DBSource_ePWMxB=ePWMxA  DBPeriodUnits=Clock cycles  DBperiodSource=Specify via dialog  REDperiod=2  FEDperiod=2  REDperiod_sec=0  FEDperiod_sec=0  LoadModeDBRED=Immediate without using shadow  LoadModeDBFED=Immediate without using shadow  adcstartModuleA=off  adcrequestEventA=First event  adcstartEventA=Digital Compare Module A Event 1 start of conversion (DCAEVT1.soc)  adcstartEventA_type2=Counter equals to period (CTR=PRD)  adcstartModuleB=off  adcrequestEventB=First event  adcstartEventB=Counter equals to zero (CTR=Zero)  adcstartEventB_type2=Counter equals to zero (CTR=Zero)  intEn=off  intPrd=First event  intSel=Counter equals to zero (CTR=Zero)  intSel_type2=Counter equals to zero (CTR=Zero)  hrpe=off  enHRPWM=off  HRPWM_LoadMode=Counter equals to period (CTR=PRD)  HRPWM_CTLMode=Duty or Period control mode  HRPWM_EDGMode=Both edge  hrpeb=off  enHRPWMB=off  HRPWM_LoadModeB=Counter equals to zero (CTR=ZERO)  HRPWM_CTLModeB=Duty or Period control mode  HRPWM_EDGModeB=Both edge  enHRDBRED=off  enHRDBFED=off  enSFO=on  enautoconv=on  chopperEnable=off  chopperFrequency=1  chopperFirstwidth=1  chopperDuty=12.5%  tripZonesource=Specify via dialog  tzselOSHT1=off  tzselOSHT2=off  tzselOSHT3=off  tzselOSHDCAEV1=off  tzselOSHDCBEV1=off  tzselCBC1=off  tzselCBC2=off  tzselCBC3=off  tzselCBCDCAEV2=off  tzselCBCDCBEV2=off  tzselOSHT4=off  tzselOSHT5=off  tzselOSHT6=off  tzselCBC4=off  tzselCBC5=off  tzselCBC6=off  enTzOstIntr=off  enTzCbcIntr=off  enTzDCAEVT1Intr=off  enTzDCAEVT2Intr=off  enTzDCBEVT1Intr=off  enTzDCBEVT2Intr=off  ePWMxAforced=No action  ePWMxBforced=No action  DCAEVT1forced=No action  DCBEVT1forced=No action  DCAEVT2forced=No action  DCBEVT2forced=No action  dcah=Trip Zone 1 input (TZ1)  dcal=Trip Zone 2 input (TZ2)  dcbh=Trip Zone 1 input (TZ1)  dcbl=Trip Zone 2 input (TZ2)  dcah_type2=GPTRIP1SEL/(TZ1)  dcal_type2=GPTRIP2SEL/(TZ2)  dcbh_type2=GPTRIP1SEL/(TZ1)  dcbl_type2=GPTRIP2SEL/(TZ2)  gendcaevt1=Event disabled  gendcaevt2=Event disabled  gendcbevt1=Event disabled  gendcbevt2=Event disabled  dcaevt1src=DCAEVT1 with sync  dcaevt2src=DCAEVT2 with sync  dcbevt1src=DCBEVT1 with sync  dcbevt2src=DCBEVT2 with sync  pulsesel=Counter equals to zero (CTR=Zero)  blankinv=off  blankoffset=0  blankwidth=0  evsrcsel=Filtered version of DCAEVT1 (DCAEVT1FILT)  encape=off
  ePWM-3 : c2802xlib/ePWM  PwmType=C2000_Type4  useModule=ePWM3  ePWMxLINKTBPRD=Not Linked  periodUnits=Clock cycles  timerSource=Specify via dialog  timerPeriod_clk=INNER_PWM  timerPeriod_sec=0.0001  tbshadow=Counter equals to zero  countingMode=Up-Down  phaseActiveEnable=Set counter to phase value specified via dialog  phaseDirection=Count up after sync  phaseActive=0  synchronizationEnable=off  dcaevt1Sync=off  dcbevt1Sync=off  synchronizationOption=Pass through (EPWMxSYNCI or SWFSYNC)  perSynchronizationOption=Counter equals to period (CTR=PRD)  clockPrescale=1  HSclockPrescale=1  enswap=off  ePWMxAStatus=on  ePWMxAactionLogic1=Do nothing  ePWMxAactionLogic2=Do nothing  ePWMxAactionLogic3=Clear  ePWMxAactionLogic4=Set  ePWMxAactionLogic5=Do nothing  ePWMxAactionLogic6=Do nothing  ePWMxACSFenable=off  ePWMxACSFvalue=Forcing disable  ePWMxASFreload=Immediate  ePWMxBStatus=off  ePWMxBactionLogic1=Do nothing  ePWMxBactionLogic2=Do nothing  ePWMxBactionLogic3=Clear  ePWMxBactionLogic4=Set  ePWMxBactionLogic5=Do nothing  ePWMxBactionLogic6=Do nothing  ePWMxBCSFenable=off  ePWMxBCSFvalue=Forcing disable  ePWMxBSFreload=Immediate  ePWNxBOutWay=off  ePWMxLINKCMPA=Not Linked  CMPAUnits=Clock cycles  CMPASource=Input port  CMPAValue_per=50  CMPAValue_clk=0  enCMPAshadow=Counter equals to zero (CTR=Zero)  ePWMxLINKCMPB=Not Linked  CMPBUnits=Clock cycles  CMPBSource=Specify via dialog  CMPBValue_per=50  CMPBValue_clk=32000  enCMPBshadow=Counter equals to zero (CTR=Zero)  ePWMxLINKCMPC=Not Linked  CMPCUnits=Clock cycles  CMPCSource=Specify via dialog  CMPCValue_per=50  CMPCValue_clk=32000  enCMPCshadow=Counter equals to zero (CTR=Zero)  ePWMxLINKCMPD=Not Linked  CMPDUnits=Clock cycles  CMPDSource=Specify via dialog  CMPDValue_per=50  CMPDValue_clk=32000  enCMPDshadow=Counter equals to zero (CTR=Zero)  enableDBePWMxA=on  enableDBePWMxB=on  enhalfcycle=off  DBpolarity=Active high complementary (AHC)  DBedgeDelay=Positive  DBSource_ePWMxA=ePWMxA  DBSource_ePWMxB=ePWMxA  DBPeriodUnits=Clock cycles  DBperiodSource=Specify via dialog  REDperiod=2  FEDperiod=2  REDperiod_sec=0  FEDperiod_sec=0  LoadModeDBRED=Immediate without using shadow  LoadModeDBFED=Immediate without using shadow  adcstartModuleA=off  adcrequestEventA=First event  adcstartEventA=Digital Compare Module A Event 1 start of conversion (DCAEVT1.soc)  adcstartEventA_type2=Counter equals to period (CTR=PRD)  adcstartModuleB=off  adcrequestEventB=First event  adcstartEventB=Counter equals to zero (CTR=Zero)  adcstartEventB_type2=Counter equals to zero (CTR=Zero)  intEn=off  intPrd=First event  intSel=Counter equals to zero (CTR=Zero)  intSel_type2=Counter equals to zero (CTR=Zero)  hrpe=off  enHRPWM=off  HRPWM_LoadMode=Counter equals to period (CTR=PRD)  HRPWM_CTLMode=Duty or Period control mode  HRPWM_EDGMode=Both edge  hrpeb=off  enHRPWMB=off  HRPWM_LoadModeB=Counter equals to zero (CTR=ZERO)  HRPWM_CTLModeB=Duty or Period control mode  HRPWM_EDGModeB=Both edge  enHRDBRED=off  enHRDBFED=off  enSFO=on  enautoconv=on  chopperEnable=off  chopperFrequency=1  chopperFirstwidth=1  chopperDuty=12.5%  tripZonesource=Specify via dialog  tzselOSHT1=off  tzselOSHT2=off  tzselOSHT3=off  tzselOSHDCAEV1=off  tzselOSHDCBEV1=off  tzselCBC1=off  tzselCBC2=off  tzselCBC3=off  tzselCBCDCAEV2=off  tzselCBCDCBEV2=off  tzselOSHT4=off  tzselOSHT5=off  tzselOSHT6=off  tzselCBC4=off  tzselCBC5=off  tzselCBC6=off  enTzOstIntr=off  enTzCbcIntr=off  enTzDCAEVT1Intr=off  enTzDCAEVT2Intr=off  enTzDCBEVT1Intr=off  enTzDCBEVT2Intr=off  ePWMxAforced=No action  ePWMxBforced=No action  DCAEVT1forced=No action  DCBEVT1forced=No action  DCAEVT2forced=No action  DCBEVT2forced=No action  dcah=Trip Zone 1 input (TZ1)  dcal=Trip Zone 2 input (TZ2)  dcbh=Trip Zone 1 input (TZ1)  dcbl=Trip Zone 2 input (TZ2)  dcah_type2=GPTRIP1SEL/(TZ1)  dcal_type2=GPTRIP2SEL/(TZ2)  dcbh_type2=GPTRIP1SEL/(TZ1)  dcbl_type2=GPTRIP2SEL/(TZ2)  gendcaevt1=Event disabled  gendcaevt2=Event disabled  gendcbevt1=Event disabled  gendcbevt2=Event disabled  dcaevt1src=DCAEVT1 with sync  dcaevt2src=DCAEVT2 with sync  dcbevt1src=DCBEVT1 with sync  dcbevt2src=DCBEVT2 with sync  pulsesel=Counter equals to zero (CTR=Zero)  blankinv=off  blankoffset=0  blankwidth=0  evsrcsel=Filtered version of DCAEVT1 (DCAEVT1FILT)  encape=off
  ePWM-4 : c2802xlib/ePWM  PwmType=C2000_Type4  useModule=ePWM4  ePWMxLINKTBPRD=Not Linked  periodUnits=Clock cycles  timerSource=Specify via dialog  timerPeriod_clk=INNER_PWM  timerPeriod_sec=0.0001  tbshadow=Counter equals to zero  countingMode=Up-Down  phaseActiveEnable=Set counter to phase value specified via dialog  phaseDirection=Count up after sync  phaseActive=0  synchronizationEnable=off  dcaevt1Sync=off  dcbevt1Sync=off  synchronizationOption=Pass through (EPWMxSYNCI or SWFSYNC)  perSynchronizationOption=Counter equals to period (CTR=PRD)  clockPrescale=1  HSclockPrescale=1  enswap=off  ePWMxAStatus=on  ePWMxAactionLogic1=Do nothing  ePWMxAactionLogic2=Do nothing  ePWMxAactionLogic3=Clear  ePWMxAactionLogic4=Set  ePWMxAactionLogic5=Do nothing  ePWMxAactionLogic6=Do nothing  ePWMxACSFenable=off  ePWMxACSFvalue=Forcing disable  ePWMxASFreload=Immediate  ePWMxBStatus=off  ePWMxBactionLogic1=Do nothing  ePWMxBactionLogic2=Do nothing  ePWMxBactionLogic3=Clear  ePWMxBactionLogic4=Set  ePWMxBactionLogic5=Do nothing  ePWMxBactionLogic6=Do nothing  ePWMxBCSFenable=off  ePWMxBCSFvalue=Forcing disable  ePWMxBSFreload=Immediate  ePWNxBOutWay=off  ePWMxLINKCMPA=Not Linked  CMPAUnits=Clock cycles  CMPASource=Input port  CMPAValue_per=50  CMPAValue_clk=0  enCMPAshadow=Counter equals to zero (CTR=Zero)  ePWMxLINKCMPB=Not Linked  CMPBUnits=Clock cycles  CMPBSource=Specify via dialog  CMPBValue_per=50  CMPBValue_clk=32000  enCMPBshadow=Counter equals to zero (CTR=Zero)  ePWMxLINKCMPC=Not Linked  CMPCUnits=Clock cycles  CMPCSource=Specify via dialog  CMPCValue_per=50  CMPCValue_clk=32000  enCMPCshadow=Counter equals to zero (CTR=Zero)  ePWMxLINKCMPD=Not Linked  CMPDUnits=Clock cycles  CMPDSource=Specify via dialog  CMPDValue_per=50  CMPDValue_clk=32000  enCMPDshadow=Counter equals to zero (CTR=Zero)  enableDBePWMxA=on  enableDBePWMxB=on  enhalfcycle=off  DBpolarity=Active high complementary (AHC)  DBedgeDelay=Positive  DBSource_ePWMxA=ePWMxA  DBSource_ePWMxB=ePWMxA  DBPeriodUnits=Clock cycles  DBperiodSource=Specify via dialog  REDperiod=2  FEDperiod=2  REDperiod_sec=0  FEDperiod_sec=0  LoadModeDBRED=Immediate without using shadow  LoadModeDBFED=Immediate without using shadow  adcstartModuleA=off  adcrequestEventA=First event  adcstartEventA=Digital Compare Module A Event 1 start of conversion (DCAEVT1.soc)  adcstartEventA_type2=Counter equals to period (CTR=PRD)  adcstartModuleB=off  adcrequestEventB=First event  adcstartEventB=Counter equals to zero (CTR=Zero)  adcstartEventB_type2=Counter equals to zero (CTR=Zero)  intEn=off  intPrd=First event  intSel=Counter equals to zero (CTR=Zero)  intSel_type2=Counter equals to zero (CTR=Zero)  hrpe=off  enHRPWM=off  HRPWM_LoadMode=Counter equals to period (CTR=PRD)  HRPWM_CTLMode=Duty or Period control mode  HRPWM_EDGMode=Both edge  hrpeb=off  enHRPWMB=off  HRPWM_LoadModeB=Counter equals to zero (CTR=ZERO)  HRPWM_CTLModeB=Duty or Period control mode  HRPWM_EDGModeB=Both edge  enHRDBRED=off  enHRDBFED=off  enSFO=on  enautoconv=on  chopperEnable=off  chopperFrequency=1  chopperFirstwidth=1  chopperDuty=12.5%  tripZonesource=Specify via dialog  tzselOSHT1=off  tzselOSHT2=off  tzselOSHT3=off  tzselOSHDCAEV1=off  tzselOSHDCBEV1=off  tzselCBC1=off  tzselCBC2=off  tzselCBC3=off  tzselCBCDCAEV2=off  tzselCBCDCBEV2=off  tzselOSHT4=off  tzselOSHT5=off  tzselOSHT6=off  tzselCBC4=off  tzselCBC5=off  tzselCBC6=off  enTzOstIntr=off  enTzCbcIntr=off  enTzDCAEVT1Intr=off  enTzDCAEVT2Intr=off  enTzDCBEVT1Intr=off  enTzDCBEVT2Intr=off  ePWMxAforced=No action  ePWMxBforced=No action  DCAEVT1forced=No action  DCBEVT1forced=No action  DCAEVT2forced=No action  DCBEVT2forced=No action  dcah=Trip Zone 1 input (TZ1)  dcal=Trip Zone 2 input (TZ2)  dcbh=Trip Zone 1 input (TZ1)  dcbl=Trip Zone 2 input (TZ2)  dcah_type2=GPTRIP1SEL/(TZ1)  dcal_type2=GPTRIP2SEL/(TZ2)  dcbh_type2=GPTRIP1SEL/(TZ1)  dcbl_type2=GPTRIP2SEL/(TZ2)  gendcaevt1=Event disabled  gendcaevt2=Event disabled  gendcbevt1=Event disabled  gendcbevt2=Event disabled  dcaevt1src=DCAEVT1 with sync  dcaevt2src=DCAEVT2 with sync  dcbevt1src=DCBEVT1 with sync  dcbevt2src=DCBEVT2 with sync  pulsesel=Counter equals to zero (CTR=Zero)  blankinv=off  blankoffset=0  blankwidth=0  evsrcsel=Filtered version of DCAEVT1 (DCAEVT1FILT)  encape=off
  ePWM-5 : c2802xlib/ePWM  PwmType=C2000_Type4  useModule=ePWM5  ePWMxLINKTBPRD=Not Linked  periodUnits=Clock cycles  timerSource=Specify via dialog  timerPeriod_clk=INNER_PWM  timerPeriod_sec=0.0001  tbshadow=Counter equals to zero  countingMode=Up-Down  phaseActiveEnable=Disable  phaseDirection=Count up after sync  phaseActive=0  synchronizationEnable=off  dcaevt1Sync=off  dcbevt1Sync=off  synchronizationOption=Counter equals to zero (CTR=Zero)  perSynchronizationOption=Counter equals to period (CTR=PRD)  clockPrescale=1  HSclockPrescale=1  enswap=off  ePWMxAStatus=on  ePWMxAactionLogic1=Do nothing  ePWMxAactionLogic2=Do nothing  ePWMxAactionLogic3=Clear  ePWMxAactionLogic4=Set  ePWMxAactionLogic5=Do nothing  ePWMxAactionLogic6=Do nothing  ePWMxACSFenable=off  ePWMxACSFvalue=Forcing disable  ePWMxASFreload=Immediate  ePWMxBStatus=off  ePWMxBactionLogic1=Do nothing  ePWMxBactionLogic2=Do nothing  ePWMxBactionLogic3=Clear  ePWMxBactionLogic4=Set  ePWMxBactionLogic5=Do nothing  ePWMxBactionLogic6=Do nothing  ePWMxBCSFenable=off  ePWMxBCSFvalue=Forcing disable  ePWMxBSFreload=Immediate  ePWNxBOutWay=off  ePWMxLINKCMPA=Not Linked  CMPAUnits=Clock cycles  CMPASource=Input port  CMPAValue_per=50  CMPAValue_clk=0  enCMPAshadow=Counter equals to zero (CTR=Zero)  ePWMxLINKCMPB=Not Linked  CMPBUnits=Clock cycles  CMPBSource=Specify via dialog  CMPBValue_per=50  CMPBValue_clk=32000  enCMPBshadow=Counter equals to zero (CTR=Zero)  ePWMxLINKCMPC=Not Linked  CMPCUnits=Clock cycles  CMPCSource=Specify via dialog  CMPCValue_per=50  CMPCValue_clk=32000  enCMPCshadow=Counter equals to zero (CTR=Zero)  ePWMxLINKCMPD=Not Linked  CMPDUnits=Clock cycles  CMPDSource=Specify via dialog  CMPDValue_per=50  CMPDValue_clk=32000  enCMPDshadow=Counter equals to zero (CTR=Zero)  enableDBePWMxA=on  enableDBePWMxB=on  enhalfcycle=on  DBpolarity=Active high complementary (AHC)  DBedgeDelay=Positive  DBSource_ePWMxA=ePWMxA  DBSource_ePWMxB=ePWMxA  DBPeriodUnits=Clock cycles  DBperiodSource=Specify via dialog  REDperiod=2  FEDperiod=2  REDperiod_sec=0  FEDperiod_sec=0  LoadModeDBRED=Immediate without using shadow  LoadModeDBFED=Immediate without using shadow  adcstartModuleA=off  adcrequestEventA=First event  adcstartEventA=Digital Compare Module A Event 1 start of conversion (DCAEVT1.soc)  adcstartEventA_type2=Counter equals to period (CTR=PRD)  adcstartModuleB=off  adcrequestEventB=First event  adcstartEventB=Counter equals to zero (CTR=Zero)  adcstartEventB_type2=Counter equals to zero (CTR=Zero)  intEn=off  intPrd=First event  intSel=Counter equals to zero (CTR=Zero)  intSel_type2=Counter equals to zero (CTR=Zero)  hrpe=off  enHRPWM=off  HRPWM_LoadMode=Counter equals to period (CTR=PRD)  HRPWM_CTLMode=Duty or Period control mode  HRPWM_EDGMode=Both edge  hrpeb=off  enHRPWMB=off  HRPWM_LoadModeB=Counter equals to zero (CTR=ZERO)  HRPWM_CTLModeB=Duty or Period control mode  HRPWM_EDGModeB=Both edge  enHRDBRED=off  enHRDBFED=off  enSFO=on  enautoconv=on  chopperEnable=off  chopperFrequency=1  chopperFirstwidth=1  chopperDuty=12.5%  tripZonesource=Specify via dialog  tzselOSHT1=off  tzselOSHT2=off  tzselOSHT3=off  tzselOSHDCAEV1=off  tzselOSHDCBEV1=off  tzselCBC1=off  tzselCBC2=off  tzselCBC3=off  tzselCBCDCAEV2=off  tzselCBCDCBEV2=off  tzselOSHT4=off  tzselOSHT5=off  tzselOSHT6=off  tzselCBC4=off  tzselCBC5=off  tzselCBC6=off  enTzOstIntr=off  enTzCbcIntr=off  enTzDCAEVT1Intr=off  enTzDCAEVT2Intr=off  enTzDCBEVT1Intr=off  enTzDCBEVT2Intr=off  ePWMxAforced=No action  ePWMxBforced=No action  DCAEVT1forced=No action  DCBEVT1forced=No action  DCAEVT2forced=No action  DCBEVT2forced=No action  dcah=Trip Zone 1 input (TZ1)  dcal=Trip Zone 2 input (TZ2)  dcbh=Trip Zone 1 input (TZ1)  dcbl=Trip Zone 2 input (TZ2)  dcah_type2=GPTRIP1SEL/(TZ1)  dcal_type2=GPTRIP2SEL/(TZ2)  dcbh_type2=GPTRIP1SEL/(TZ1)  dcbl_type2=GPTRIP2SEL/(TZ2)  gendcaevt1=Event disabled  gendcaevt2=Event disabled  gendcbevt1=Event disabled  gendcbevt2=Event disabled  dcaevt1src=DCAEVT1 with sync  dcaevt2src=DCAEVT2 with sync  dcbevt1src=DCBEVT1 with sync  dcbevt2src=DCBEVT2 with sync  pulsesel=Counter equals to zero (CTR=Zero)  blankinv=off  blankoffset=0  blankwidth=0  evsrcsel=Filtered version of DCAEVT1 (DCAEVT1FILT)  encape=off
  ePWM-6 : c2802xlib/ePWM  PwmType=C2000_Type4  useModule=ePWM6  ePWMxLINKTBPRD=Not Linked  periodUnits=Clock cycles  timerSource=Specify via dialog  timerPeriod_clk=INNER_PWM  timerPeriod_sec=0.0001  tbshadow=Counter equals to zero  countingMode=Up-Down  phaseActiveEnable=Disable  phaseDirection=Count down after sync  phaseActive=0  synchronizationEnable=off  dcaevt1Sync=off  dcbevt1Sync=off  synchronizationOption=Counter equals to zero (CTR=Zero)  perSynchronizationOption=Counter equals to period (CTR=PRD)  clockPrescale=1  HSclockPrescale=1  enswap=off  ePWMxAStatus=on  ePWMxAactionLogic1=Do nothing  ePWMxAactionLogic2=Do nothing  ePWMxAactionLogic3=Clear  ePWMxAactionLogic4=Set  ePWMxAactionLogic5=Do nothing  ePWMxAactionLogic6=Do nothing  ePWMxACSFenable=off  ePWMxACSFvalue=Forcing disable  ePWMxASFreload=Immediate  ePWMxBStatus=off  ePWMxBactionLogic1=Do nothing  ePWMxBactionLogic2=Do nothing  ePWMxBactionLogic3=Clear  ePWMxBactionLogic4=Set  ePWMxBactionLogic5=Do nothing  ePWMxBactionLogic6=Do nothing  ePWMxBCSFenable=off  ePWMxBCSFvalue=Forcing disable  ePWMxBSFreload=Immediate  ePWNxBOutWay=off  ePWMxLINKCMPA=Not Linked  CMPAUnits=Clock cycles  CMPASource=Input port  CMPAValue_per=50  CMPAValue_clk=0  enCMPAshadow=Counter equals to zero (CTR=Zero)  ePWMxLINKCMPB=Not Linked  CMPBUnits=Clock cycles  CMPBSource=Specify via dialog  CMPBValue_per=50  CMPBValue_clk=32000  enCMPBshadow=Counter equals to zero (CTR=Zero)  ePWMxLINKCMPC=Not Linked  CMPCUnits=Clock cycles  CMPCSource=Specify via dialog  CMPCValue_per=50  CMPCValue_clk=32000  enCMPCshadow=Counter equals to zero (CTR=Zero)  ePWMxLINKCMPD=Not Linked  CMPDUnits=Clock cycles  CMPDSource=Specify via dialog  CMPDValue_per=50  CMPDValue_clk=32000  enCMPDshadow=Counter equals to zero (CTR=Zero)  enableDBePWMxA=on  enableDBePWMxB=on  enhalfcycle=on  DBpolarity=Active high complementary (AHC)  DBedgeDelay=Positive  DBSource_ePWMxA=ePWMxA  DBSource_ePWMxB=ePWMxA  DBPeriodUnits=Clock cycles  DBperiodSource=Specify via dialog  REDperiod=2  FEDperiod=2  REDperiod_sec=0  FEDperiod_sec=0  LoadModeDBRED=Immediate without using shadow  LoadModeDBFED=Immediate without using shadow  adcstartModuleA=off  adcrequestEventA=First event  adcstartEventA=Digital Compare Module A Event 1 start of conversion (DCAEVT1.soc)  adcstartEventA_type2=Counter equals to period (CTR=PRD)  adcstartModuleB=off  adcrequestEventB=First event  adcstartEventB=Counter equals to zero (CTR=Zero)  adcstartEventB_type2=Counter equals to zero (CTR=Zero)  intEn=off  intPrd=First event  intSel=Counter equals to zero (CTR=Zero)  intSel_type2=Counter equals to zero (CTR=Zero)  hrpe=off  enHRPWM=off  HRPWM_LoadMode=Counter equals to period (CTR=PRD)  HRPWM_CTLMode=Duty or Period control mode  HRPWM_EDGMode=Both edge  hrpeb=off  enHRPWMB=off  HRPWM_LoadModeB=Counter equals to zero (CTR=ZERO)  HRPWM_CTLModeB=Duty or Period control mode  HRPWM_EDGModeB=Both edge  enHRDBRED=off  enHRDBFED=off  enSFO=on  enautoconv=on  chopperEnable=off  chopperFrequency=1  chopperFirstwidth=1  chopperDuty=12.5%  tripZonesource=Specify via dialog  tzselOSHT1=off  tzselOSHT2=off  tzselOSHT3=off  tzselOSHDCAEV1=off  tzselOSHDCBEV1=off  tzselCBC1=off  tzselCBC2=off  tzselCBC3=off  tzselCBCDCAEV2=off  tzselCBCDCBEV2=off  tzselOSHT4=off  tzselOSHT5=off  tzselOSHT6=off  tzselCBC4=off  tzselCBC5=off  tzselCBC6=off  enTzOstIntr=off  enTzCbcIntr=off  enTzDCAEVT1Intr=off  enTzDCAEVT2Intr=off  enTzDCBEVT1Intr=off  enTzDCBEVT2Intr=off  ePWMxAforced=No action  ePWMxBforced=No action  DCAEVT1forced=No action  DCBEVT1forced=No action  DCAEVT2forced=No action  DCBEVT2forced=No action  dcah=Trip Zone 1 input (TZ1)  dcal=Trip Zone 2 input (TZ2)  dcbh=Trip Zone 1 input (TZ1)  dcbl=Trip Zone 2 input (TZ2)  dcah_type2=GPTRIP1SEL/(TZ1)  dcal_type2=GPTRIP2SEL/(TZ2)  dcbh_type2=GPTRIP1SEL/(TZ1)  dcbl_type2=GPTRIP2SEL/(TZ2)  gendcaevt1=Event disabled  gendcaevt2=Event disabled  gendcbevt1=Event disabled  gendcbevt2=Event disabled  dcaevt1src=DCAEVT1 with sync  dcaevt2src=DCAEVT2 with sync  dcbevt1src=DCBEVT1 with sync  dcbevt2src=DCBEVT2 with sync  pulsesel=Counter equals to zero (CTR=Zero)  blankinv=off  blankoffset=0  blankwidth=0  evsrcsel=Filtered version of DCAEVT1 (DCAEVT1FILT)  encape=off
  voltage divider : Gain  Gain=(6*560)/((43*39)/(43+39))  ParamDataTypeStr=Inherit: Inherit from 'Gain'  OutDataTypeStr=single
  voltage divider1 : Gain  Gain=(6*560)/((43*39)/(43+39))  ParamDataTypeStr=Inherit: Inherit from 'Gain'  OutDataTypeStr=single
  Out1 : Outport  VectorParamsAs1DForOutWhenUnconnected=off
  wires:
  Rate Transition1/1 -> Out1/1
  Pack data for CAN/1(Output) -> Rate Transition1/1
  Normalize1/1 -> [Theta]
  Data Store Read/1 -> Normalize1/1
  Data Store Read1/1 -> Normalize1/2
  In1/1 -> Demux/1
  RED LED/1 -> RD_LED_GPIO/1
  GREEN LED/1 -> GRN_LED_GPIO1/1
  Demux/1 -> [PRECHARGE_OFF], [GRID_ON]
  [GRID_ON] -> Data Type Conversion3/1
  Data Type Conversion3/1 -> Digital Output6/1
  Data Type Conversion4/1 -> Digital Output1/1
  [PRECHARGE_OFF] -> Data Type Conversion4/1
  Newinv1/3(Id) -> [I_d_ADC]
  ADC4/1 -> Newinv1/1(A4)
  Newinv1/2(Vq) -> [V_q_ADC]
  [Theta] -> Newinv1/7(theta)
  Newinv1/4(Iq) -> [I_q_ADC]
  Newinv2/1(Vd) -> [V_d_ADC_EXT]
  Newinv2/4(Iq) -> [I_q_ADC_EXT]
  ADC1/1 -> Newinv1/4(B0)
  Newinv1/1(Vd) -> [V_d_ADC]
  [Theta] -> Newinv2/7(theta)
  ADC2/1 -> Newinv1/5(B1)
  Newinv2/2(Vq) -> [V_q_ADC_EXT]
  Newinv2/3(Id) -> [I_d_ADC_EXT]
  ADC3/1 -> Newinv1/6(B2)
  ADCD2/1 -> Data Type Conversion10/1
  ADCD0/1 -> Data Type Conversion9/1
  voltage divider1/1 -> Data Store Write2/1, Gain2/1
  Convert ADC [0 4095] to voltage [0 3.3] V1/1 -> voltage divider1/1
  Data Type Conversion10/1 -> Convert ADC [0 4095] to voltage [0 3.3] V1/1
  Data Type Conversion9/1 -> Convert ADC [0 4095] to voltage [0 3.3] V/1
  ADCD1/1 -> Data Store Write/1
  Gain3/1 -> Subtract/1, [Vdc_P]
  [OnOff] -> Data Type Conversion/1
  Data Type Conversion/1 -> InvPark/SVGen + ePWM scaling/1(On/Off)
  Gain/1 -> InvPark/SVGen + ePWM scaling/2("u_d ")
  Gain7/1 -> InvPark/SVGen + ePWM scaling/3("u_q ")
  [Theta] -> InvPark/SVGen + ePWM scaling/4(Theta)
  InvPark/SVGen + ePWM scaling/1(ePWM_12) -> ePWM-12/1
  InvPark/SVGen + ePWM scaling/2(ePWM_11) -> ePWM-11/1
  InvPark/SVGen + ePWM scaling/3(ePWM_10) -> ePWM-10/1
  IQN to Float1/1 -> Speed IIR filter1/1(Speed)
  [Ud_ref] -> Data Type Conversion1/1
  Demux/2 -> [OnOff]
  Demux/3 -> [Ud_ref]
  Data Type Conversion1/1 -> Gain/1
  Data Type Conversion11/1 -> Gain7/1
  IQN to Float5/1 -> Speed IIR filter/1(Speed)
  InvPark/SVGen + ePWM scaling/4(ePWM_6) -> ePWM-6/1
  InvPark/SVGen + ePWM scaling/5(ePWM_5) -> ePWM-5/1
  InvPark/SVGen + ePWM scaling/6(ePWM_4) -> ePWM-4/1
  InvPark/SVGen + ePWM scaling/7(ePWM_3) -> ePWM-3/1
  InvPark/SVGen + ePWM scaling/8("ePWM_2 ") -> "ePWM-2 "/1
  InvPark/SVGen + ePWM scaling/9(ePWM_1) -> "ePWM-1 "/1
  Convert ADC [0 4095] to voltage [0 3.3] V/1 -> voltage divider/1
  voltage divider/1 -> Data Store Write1/1, Gain3/1
  Data Type Conversion6/1 -> Pack data for CAN/1(In1)
  Data Type Conversion5/1 -> Pack data for CAN/2(In2)
  Data Type Conversion7/1 -> Pack data for CAN/3(In3)
  Data Type Conversion8/1 -> Pack data for CAN/4(In4)
  Speed IIR filter/1(Filtered speed) -> Gain1/1
  [Uq_ref] -> Data Type Conversion11/1
  Demux/4 -> [Uq_ref]
  Speed IIR filter2/1(Filtered speed) -> Gain5/1
  Speed IIR filter3/1(Filtered speed) -> Gain6/1
  Gain2/1 -> Subtract/2, [Vdc_N]
  Speed IIR filter1/1(Filtered speed) -> Gain4/1
  ADC5/1 -> Newinv1/2(A5)
  ADC6/1 -> Newinv1/3(A6)
  Gain1/1 -> Data Type Conversion6/1
  Gain4/1 -> Data Type Conversion5/1
  Gain5/1 -> Data Type Conversion7/1
  Gain6/1 -> Data Type Conversion8/1
  IQN to Float2/1 -> Speed IIR filter2/1(Speed)
  IQN to Float3/1 -> Speed IIR filter3/1(Speed)
  ADC12/1 -> Newinv2/1(A4)
  ADC13/1 -> Newinv2/2(A5)
  ADC19/1 -> Newinv2/3(A6)
  ADC14/1 -> Newinv2/4(B0)
  ADC15/1 -> Newinv2/5(B1)
  ADC16/1 -> Newinv2/6(B2)
  [I_q_ADC_EXT] -> IQN to Float3/1
  [I_d_ADC_EXT] -> IQN to Float2/1
  [V_d_ADC_EXT] -> IQN to Float5/1
  [V_q_ADC_EXT] -> IQN to Float1/1
